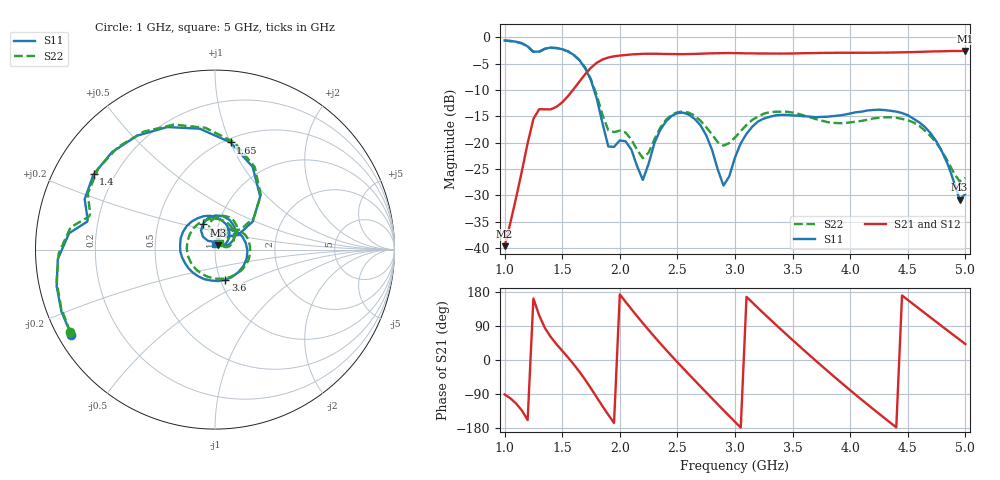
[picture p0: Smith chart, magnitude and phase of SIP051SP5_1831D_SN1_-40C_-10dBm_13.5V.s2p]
# GHz  S  dB  R  50
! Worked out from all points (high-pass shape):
!   81 points, 1 GHz to 5 GHz, reference 50 ohm
!   highest |S21| = -2.61 dB at 5 GHz (marker M1); lowest = -39.7 dB at 1 GHz (marker M2)
!   |S21| within 3 dB of the highest: 1.76 GHz to end of sweep
!   lowest |S11| = -30.9 dB at 4.95 GHz (marker M3), VSWR 1.06, Z = 51.6 + j2.4 ohm
!   |S11| at or under -10 dB: 1.776 GHz to end of sweep
!   |S22| runs from -27.4 to -0.6 dB; largest |S21 - S12| = 0.0021
!   S11 on the Smith chart (normalised r, x): 1 GHz: 0.04, -0.27; 1.4 GHz: 0.12, +0.28; 1.65 GHz: 0.53, +1.00; 2.4 GHz: 0.84, +0.25; 3.6 GHz: 1.06, -0.37; 5 GHz: 1.00, +0.07
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1  -0.62 -149.4  -39.68 -90.8  -39.60 -90.3  -0.64 -150.4
1.25  -2.75 167.6  -15.51 162.4  -15.51 162.5  -2.79 165.2
1.4  -1.98 148.1  -13.71 61.0  -13.71 61.1  -2.03 145.3
1.65  -4.39 81.7  -8.41 -31.1  -8.41 -31.1  -4.33 79.8
1.7  -5.91 65.6  -7.01 -52.2  -7.02 -52.2  -5.83 64.4
1.85  -16.38 32.4  -4.23 -122.0  -4.23 -122.0  -14.78 38.0
2  -19.60 78.1  -3.49 173.3  -3.48 173.3  -17.75 66.5
2.2  -27.10 98.4  -3.16 97.2  -3.17 97.3  -22.96 79.6
2.35  -17.64 126.3  -3.17 44.2  -3.16 44.3  -17.23 103.8
2.4  -16.01 115.0  -3.19 27.3  -3.18 27.3  -15.71 96.7
2.55  -14.33 76.5  -3.22 -21.9  -3.20 -21.9  -14.09 66.7
2.75  -18.63 27.9  -3.10 -85.5  -3.09 -85.5  -17.08 34.8
2.9  -28.18 43.5  -3.03 -132.5  -3.02 -132.5  -20.60 43.2
3  -22.84 80.5  -3.03 -163.2  -3.02 -163.2  -19.05 55.2
3.3  -15.13 12.3  -3.10 108.6  -3.10 108.6  -14.24 16.2
3.6  -15.01 -71.3  -3.04 25.4  -3.05 25.4  -14.88 -49.9
3.7  -15.20 -97.4  -3.02 -1.5  -3.01 -1.6  -15.55 -76.6
4  -14.49 -166.9  -2.96 -79.7  -2.96 -79.8  -16.17 -167.6
4.35  -13.98 119.2  -2.92 -165.9  -2.92 -165.8  -15.21 97.2
4.7  -18.29 48.7  -2.71 111.6  -2.71 111.6  -18.84 25.3
4.95  -30.87 54.2  -2.63 53.5  -2.62 53.5  -27.37 33.3
5  -29.75 90.0  -2.61 42.0  -2.61 41.9  -26.72 51.3
